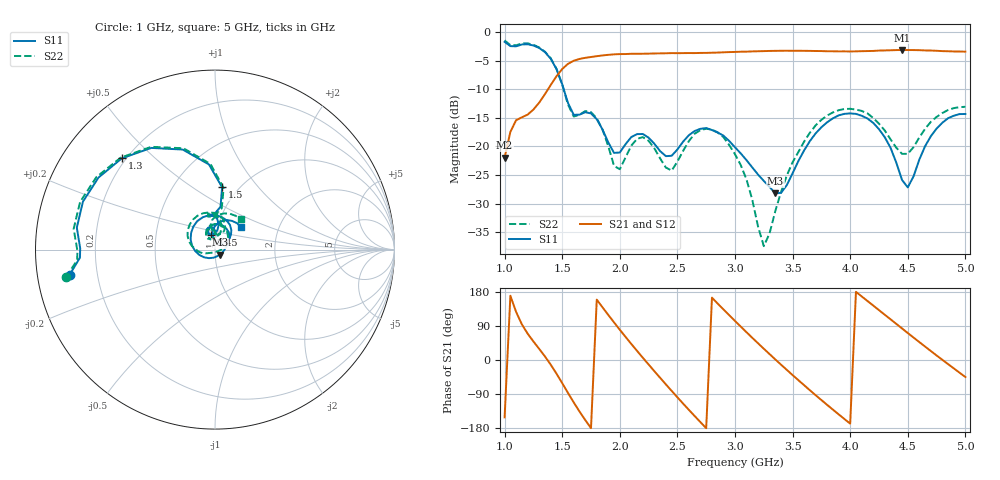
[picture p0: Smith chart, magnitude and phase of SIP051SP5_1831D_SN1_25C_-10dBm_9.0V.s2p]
# GHz  S  dB  R  50
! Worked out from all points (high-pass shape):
!   81 points, 1 GHz to 5 GHz, reference 50 ohm
!   highest |S21| = -3.13 dB at 4.45 GHz (marker M1); lowest = -22.0 dB at 1 GHz (marker M2)
!   |S21| within 3 dB of the highest: 1.518 GHz to end of sweep
!   lowest |S11| = -28.2 dB at 3.35 GHz (marker M3), VSWR 1.08, Z = 52.7 - j2.92 ohm
!   |S11| at or under -10 dB: 1.513 GHz to end of sweep
!   |S22| runs from -37.5 to -1.5 dB; largest |S21 - S12| = 0.002
!   S11 on the Smith chart (normalised r, x): 1 GHz: 0.10, -0.09; 1.3 GHz: 0.18, +0.40; 1.5 GHz: 0.84, +0.67; 2.45 GHz: 0.95, +0.15; 5 GHz: 1.29, +0.34
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1  -1.70 -170.2  -21.99 -151.4  -22.02 -151.8  -1.46 -169.5
1.1  -2.49 179.5  -15.42 126.7  -15.42 127.0  -2.31 -179.6
1.3  -2.77 135.6  -12.35 29.4  -12.34 29.5  -2.69 135.7
1.5  -9.14 83.5  -6.46 -61.0  -6.46 -60.9  -9.21 82.0
1.6  -14.48 93.8  -5.01 -111.9  -5.01 -111.9  -14.78 93.0
1.7  -14.01 100.3  -4.50 -158.4  -4.51 -158.4  -13.82 100.5
1.85  -17.06 81.5  -4.08 138.9  -4.08 138.9  -17.06 74.4
2  -21.07 109.8  -3.85 79.8  -3.85 79.9  -24.00 110.7
2.2  -17.83 99.9  -3.79 5.9  -3.79 5.9  -18.38 103.6
2.35  -20.83 90.8  -3.72 -47.0  -3.72 -46.9  -22.11 87.2
2.45  -21.64 105.1  -3.68 -81.5  -3.70 -81.5  -24.23 112.6
2.75  -16.80 78.8  -3.64 -180.0  -3.63 -179.9  -16.92 88.9
3  -20.16 35.6  -3.47 103.0  -3.46 103.1  -21.37 33.1
3.25  -26.04 -5.9  -3.33 29.7  -3.32 29.8  -37.46 -68.4
3.35  -28.23 -45.5  -3.28 1.5  -3.29 1.6  -31.31 -139.0
3.55  -22.57 -144.6  -3.27 -53.2  -3.27 -53.3  -20.99 -171.8
3.7  -17.73 170.1  -3.31 -92.9  -3.31 -92.8  -16.32 162.2
4.05  -14.31 89.0  -3.37 179.9  -3.37 179.9  -13.56 98.9
4.35  -20.23 36.5  -3.18 107.5  -3.18 107.4  -18.76 64.0
4.45  -25.88 44.9  -3.13 83.3  -3.13 83.3  -21.31 75.6
4.75  -16.88 85.7  -3.27 11.9  -3.28 12.1  -14.85 90.5
5  -14.33 41.2  -3.42 -44.9  -3.42 -44.9  -13.07 50.1
